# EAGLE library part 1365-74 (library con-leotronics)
DUAL ROW STRAIGHT HEADER 1364 SERIES. 1.27mm x 1.27mm. Without Fixing Post. SMT Source: http://www.leotronics.co.uk/Conexcon/Data%20Sheets/sec.%20A/1364ing.pdf
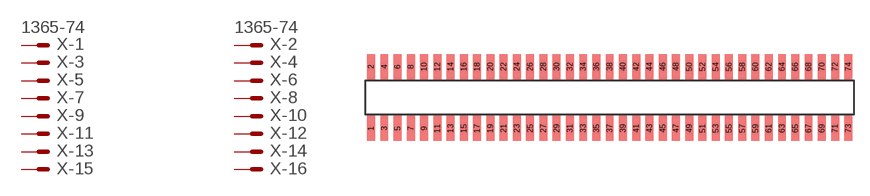
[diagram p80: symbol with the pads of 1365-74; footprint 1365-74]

Designator prefix X; gates -1=MVAL -2=MVAL -3=M -4=M -5=M -6=M -7=M -8=M -9=M -10=M -11=M -12=M -13=M -14=M -15=M -16=M -17=M -18=M -19=M -20=M -21=M -22=M -23=M -24=M -25=M -26=M -27=M -28=M -29=M -30=M -31=M -32=M -33=M -34=M -35=M -36=M -37=M -38=M -39=M -40=M -41=M -42=M -43=M -44=M -45=M -46=M -47=M -48=M -49=M -50=M -51=M -52=M -53=M -54=M -55=M -56=M -57=M -58=M -59=M -60=M -61=M -62=M -63=M -64=M -65=M -66=M -67=M -68=M -69=M -70=M -71=M -72=M -73=M -74=M

## 1365-74 (OC_FARNELL: unknown; OC_NEWARK: unknown)  [1365-74]
1  -1:S  pas
2  -2:S  pas
3  -3:S  pas
4  -4:S  pas
5  -5:S  pas
6  -6:S  pas
7  -7:S  pas
8  -8:S  pas
9  -9:S  pas
10  -10:S  pas
11  -11:S  pas
12  -12:S  pas
13  -13:S  pas
14  -14:S  pas
15  -15:S  pas
16  -16:S  pas
17  -17:S  pas
18  -18:S  pas
19  -19:S  pas
20  -20:S  pas
21  -21:S  pas
22  -22:S  pas
23  -23:S  pas
24  -24:S  pas
25  -25:S  pas
26  -26:S  pas
27  -27:S  pas
28  -28:S  pas
29  -29:S  pas
30  -30:S  pas
31  -31:S  pas
32  -32:S  pas
33  -33:S  pas
34  -34:S  pas
35  -35:S  pas
36  -36:S  pas
37  -37:S  pas
38  -38:S  pas
39  -39:S  pas
40  -40:S  pas
41  -41:S  pas
42  -42:S  pas
43  -43:S  pas
44  -44:S  pas
45  -45:S  pas
46  -46:S  pas
47  -47:S  pas
48  -48:S  pas
49  -49:S  pas
50  -50:S  pas
51  -51:S  pas
52  -52:S  pas
53  -53:S  pas
54  -54:S  pas
55  -55:S  pas
56  -56:S  pas
57  -57:S  pas
58  -58:S  pas
59  -59:S  pas
60  -60:S  pas
61  -61:S  pas
62  -62:S  pas
63  -63:S  pas
64  -64:S  pas
65  -65:S  pas
66  -66:S  pas
67  -67:S  pas
68  -68:S  pas
69  -69:S  pas
70  -70:S  pas
71  -71:S  pas
72  -72:S  pas
73  -73:S  pas
74  -74:S  pas

## Footprint 1365-74 (pad centres in mm)
DUAL ROW STRAIGHT HEADER 1364 SERIES. 1.27mm x 1.27mm. Without Fixing Post. SMT Source: http://www.leotronics.co.uk/Conexcon/Data%20Sheets/sec.%20A/1364ing.pdf
smd 0.76 x 2.4: 1 -22.86,-2.95; 2 -22.86,2.95; 3 -21.59,-2.95; 4 -21.59,2.95; 5 -20.32,-2.95; 6 -20.32,2.95; 7 -19.05,-2.95; 8 -19.05,2.95; 9 -17.78,-2.95; 10 -17.78,2.95; 11 -16.51,-2.95; 12 -16.51,2.95; 13 -15.24,-2.95; 14 -15.24,2.95; 15 -13.97,-2.95; 16 -13.97,2.95; 17 -12.7,-2.95; 18 -12.7,2.95; 19 -11.43,-2.95; 20 -11.43,2.95; 21 -10.16,-2.95; 22 -10.16,2.95; 23 -8.89,-2.95; 24 -8.89,2.95; 25 -7.62,-2.95; 26 -7.62,2.95; 27 -6.35,-2.95; 28 -6.35,2.95; 29 -5.08,-2.95; 30 -5.08,2.95; 31 -3.81,-2.95; 32 -3.81,2.95; 33 -2.54,-2.95; 34 -2.54,2.95; 35 -1.27,-2.95; 36 -1.27,2.95; 37 0,-2.95; 38 0,2.95; 39 1.27,-2.95; 40 1.27,2.95; 41 2.54,-2.95; 42 2.54,2.95; 43 3.81,-2.95; 44 3.81,2.95; 45 5.08,-2.95; 46 5.08,2.95; 47 6.35,-2.95; 48 6.35,2.95; 49 7.62,-2.95; 50 7.62,2.95; 51 8.89,-2.95; 52 8.89,2.95; 53 10.16,-2.95; 54 10.16,2.95; 55 11.43,-2.95; 56 11.43,2.95; 57 12.7,-2.95; 58 12.7,2.95; 59 13.97,-2.95; 60 13.97,2.95; 61 15.24,-2.95; 62 15.24,2.95; 63 16.51,-2.95; 64 16.51,2.95; 65 17.78,-2.95; 66 17.78,2.95; 67 19.05,-2.95; 68 19.05,2.95; 69 20.32,-2.95; 70 20.32,2.95; 71 21.59,-2.95; 72 21.59,2.95; 73 22.86,-2.95; 74 22.86,2.95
